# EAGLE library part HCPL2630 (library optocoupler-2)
HEWLETT PACKARD OPTO COUPLER
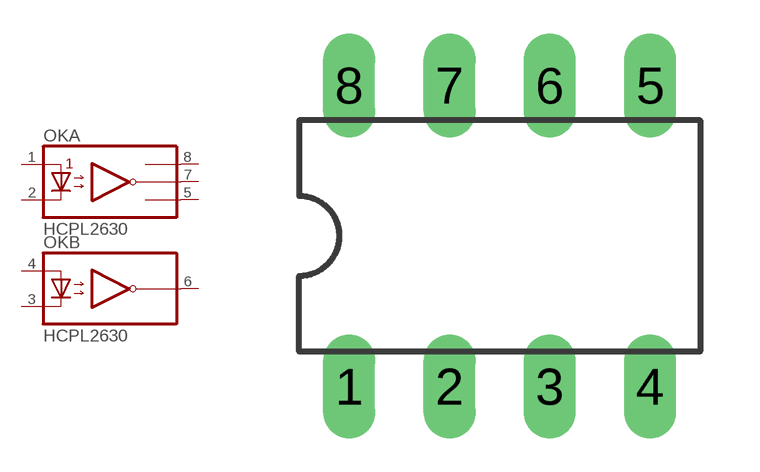
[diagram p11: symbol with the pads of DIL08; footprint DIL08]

Designator prefix OK; gates A=2630 B=2630A

## HCPL2630  [DIL08]
1  A:A1  pas
2  A:C1  pas
3  B:C2  pas
4  B:A2  pas
5  A:GND  pas
6  B:VO2  pas
7  A:VO1  pas
8  A:VCC  pas

## Footprint DIL08 (pad centres in mm)
Dual In Line Package
drill 0.813 long: 1 -3.81,-3.81; 2 -1.27,-3.81; 3 1.27,-3.81; 4 3.81,-3.81; 5 3.81,3.81; 6 1.27,3.81; 7 -1.27,3.81; 8 -3.81,3.81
